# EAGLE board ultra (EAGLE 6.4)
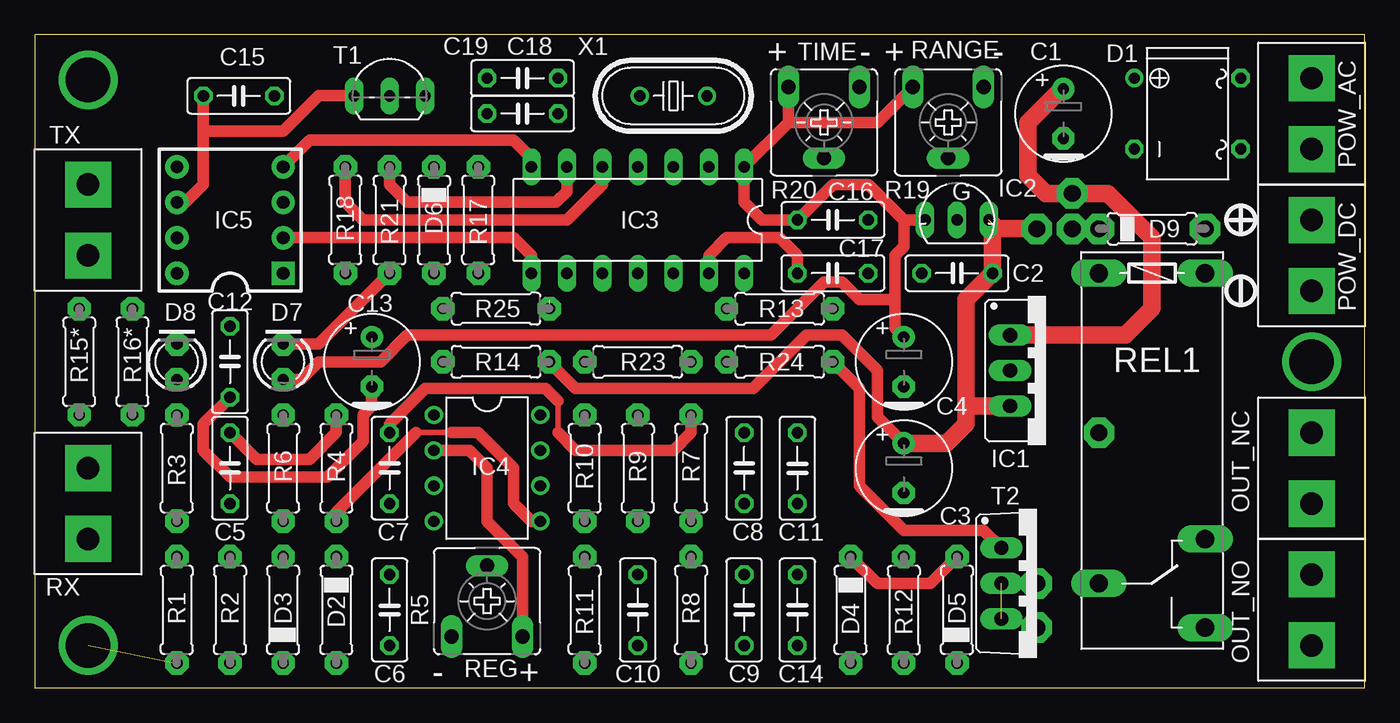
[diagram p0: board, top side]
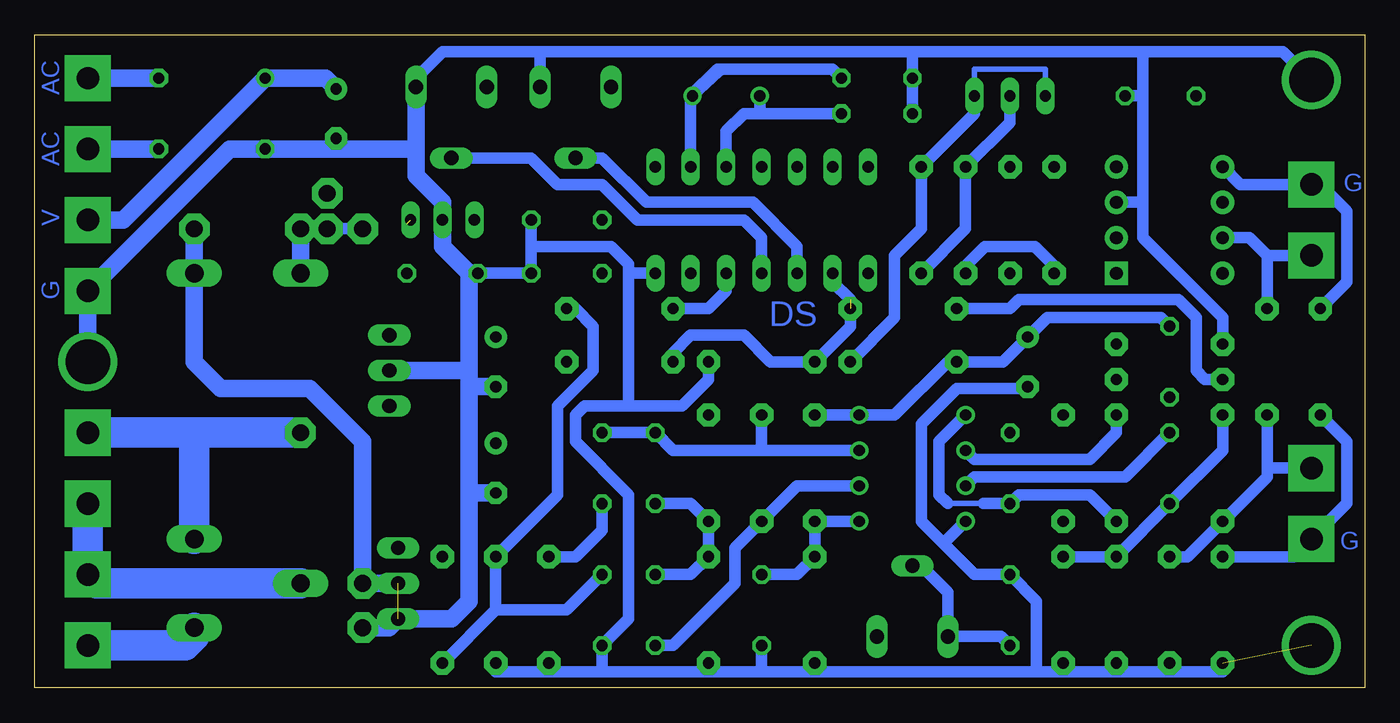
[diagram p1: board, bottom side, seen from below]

Size 95.23 x 46.79 mm. Coordinates in mm from the lower left corner, seen from the top.
Outline: 0,0 95.23,0 95.23,46.79 0,46.79 0,0
Copper layers (1*16): Top 0.035mm / dielectric 1.5mm / Bottom 0.035mm
Design rules "default": minimum track width 10mil, minimum drill 24mil, track to track 8mil, track to pad 8mil, pad to pad 8mil, via to via 8mil, smd to smd 8mil, copper to edge 40mil, drill to drill 8mil, minimum pad ring 10mil, minimum via ring 8mil, stop-mask expansion 4mil, vias tented up to drill 0mil, thermal gap 10mil

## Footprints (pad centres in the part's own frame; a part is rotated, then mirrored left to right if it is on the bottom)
E2,5-7 = drill 0.813 pad 1.6: + -1.778,0 | drill 0.813 pad 1.6 octagon: - 1.778,0
C050-025X075 = drill 0.813 octagon: 1 -2.54,0; 2 2.54,0
B-DIL = drill 0.813: + -2.54,-3.81 | drill 0.813 octagon: - 2.54,-3.81; AC1 2.54,3.81; AC2 -2.54,3.81
0207/7 = drill 0.813 pad 1.676 octagon: 1 -3.81,0; 2 3.81,0
LED3MM = drill 0.813 pad 1.676 octagon: A -1.27,0; K 1.27,0
78XXS = drill 1.016 long: GND 0,-2.54; IN -2.54,-2.54; OUT 2.54,-2.54
78LXX = drill 0.813 pad 1.27 long: GND 0,0; IN 2.286,0; OUT -2.286,0
DIL14 = drill 0.813 long: 1 -7.62,-3.81; 2 -5.08,-3.81; 3 -2.54,-3.81; 4 0,-3.81; 5 2.54,-3.81; 6 5.08,-3.81; 7 7.62,-3.81; 8 7.62,3.81; 9 5.08,3.81; 10 2.54,3.81; 11 0,3.81; 12 -2.54,3.81; 13 -5.08,3.81; 14 -7.62,3.81
DIL08 = drill 0.813 pad 1.27: 1 -3.81,-3.81; 2 -1.27,-3.81; 3 1.27,-3.81; 4 3.81,-3.81; 5 3.81,3.81; 6 1.27,3.81; 7 -1.27,3.81; 8 -3.81,3.81
MC33152 = drill 0.9 pad 1.676 square: 1 -3.81,-3.81 | drill 0.9 pad 1.676: 2 -1.27,-3.81; 3 1.27,-3.81; 4 3.81,-3.81; 5 3.81,3.81; 6 1.27,3.81; 7 -1.27,3.81; 8 -3.81,3.81
ARK2/500 = drill 1.6 pad 3.302 square: 1 -2.54,0; 2 2.54,0
CA6V = drill 1.016 long: A -2.54,-2.54; E 2.54,-2.54; S 0,2.54
G6RW = drill 1.321 long: 1 -12.7,-3.81; 2 -12.7,3.81; O 6.35,3.81; P 9.525,-3.81; S 12.7,3.81
TO92-EBC = drill 0.813 long: B 0,-1.27; C -2.54,-1.27; E 2.54,-1.27
TO220BV = drill 1.016 long: D 0,-2.54; G -2.54,-2.54; S 2.54,-2.54
HC49U70 = drill 0.813: 1 -2.413,0; 2 2.413,0

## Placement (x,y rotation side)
C1  220uF  [E2,5-7]  73.66,41.15 270 top
C2  100nF  [C050-025X075]  66.04,29.72 0 top
C3  100uF  [E2,5-7]  62.23,15.75 270 top
C4  100uF  [E2,5-7]  62.23,23.37 270 top
C5  10nF  [C050-025X075]  13.97,15.75 90 top
C6  100nF  [C050-025X075]  25.4,5.59 270 top
C7  100nF  [C050-025X075]  25.4,15.75 90 top
C8  1nF  [C050-025X075]  50.8,15.75 90 top
C9  1nF  [C050-025X075]  50.8,5.59 90 top
C10  100nF  [C050-025X075]  43.18,5.59 90 top
C11  100nF  [C050-025X075]  54.61,15.75 270 top
C12  100nF  [C050-025X075]  13.97,23.37 90 top
C13  100uF  [E2,5-7]  24.13,23.37 270 top
C14  100nF  [C050-025X075]  54.61,5.59 90 top
C15  100nF  [C050-025X075]  14.61,42.42 180 top
C16  100nF  [C050-025X075]  57.15,33.53 180 top
C17  100nF  [C050-025X075]  57.15,29.72 180 top
C18  10pF  [C050-025X075]  34.92,41.15 180 top
C19  10pF  [C050-025X075]  34.92,43.69 180 top
D1  [B-DIL]  82.55,41.15 270 top
D2  BAT43  [0207/7]  21.59,5.59 90 top
D3  BAT43  [0207/7]  17.78,5.59 90 top
D4  BAT43  [0207/7]  58.42,5.59 90 top
D5  BAT43  [0207/7]  66.04,5.59 90 top
D6  DZ9V1  [0207/7]  28.57,33.53 270 top
D7  [LED3MM]  17.78,23.37 90 top
D8  [LED3MM]  10.16,23.37 90 top
D9  BAT43  [0207/7]  80.01,32.89 180 top
IC1  LM2940-12  [78XXS]  72.39,22.73 270 top
IC2  78L05  [78LXX]  66.04,33.53 0 top
IC3  ATTINY24  [DIL14]  43.18,33.53 180 top
IC4  TL072  [DIL08]  32.38,15.75 270 top
IC5  MC33152  [MC33152]  13.97,33.53 90 top
OUT_NC  ARK2ARK2/500  [ARK2/500]  91.44,15.75 90 top
OUT_NO  ARK2ARK2/500  [ARK2/500]  91.44,5.59 90 top
POW_AC  [ARK2/500]  91.44,41.15 270 top
POW_DC  ARK2ARK2/500  [ARK2/500]  91.44,30.99 270 top
R1  100R  [0207/7]  10.16,5.59 90 top
R2  1M  [0207/7]  13.97,5.59 90 top
R3  2k  [0207/7]  10.16,15.75 270 top
R4  1M  [0207/7]  21.59,15.75 270 top
R5  100k  [CA6V]  32.38,6.22 0 top
R6  1M  [0207/7]  17.78,15.75 270 top
R7  510R  [0207/7]  46.99,15.75 270 top
R8  510R  [0207/7]  46.99,5.59 90 top
R9  68k  [0207/7]  43.18,15.75 90 top
R10  2k  [0207/7]  39.37,15.75 90 top
R11  2k  [0207/7]  39.37,5.59 90 top
R12  2k  [0207/7]  62.23,5.59 90 top
R13  10k  [0207/7]  53.34,27.18 0 top
R14  100R  [0207/7]  33.02,23.37 180 top
R15*  0R  [0207/7]  3.18,23.37 90 top
R16*  0R  [0207/7]  6.99,23.37 90 top
R17  10k  [0207/7]  31.75,33.53 270 top
R18  2k  [0207/7]  22.23,33.53 90 top
R19  100k  [CA6V]  65.41,40.51 180 top
R20  100k  [CA6V]  56.51,40.51 180 top
R21  2k  [0207/7]  25.4,33.53 90 top
R23  10k  [0207/7]  43.18,23.37 0 top
R24  100R  [0207/7]  53.34,23.37 0 top
R25  2k  [0207/7]  33.02,27.18 0 top
REL1  JQX68-12V  [G6RW]  80.01,17.02 270 top
RX  RX  [ARK2/500]  3.81,13.21 270 top
T1  BC557  [TO92-EBC]  25.4,43.69 0 top
T2  IRL540  [TO220BV]  71.76,7.49 270 top
TX  TX  [ARK2/500]  3.81,33.53 90 top
X1  16MHz  [HC49U70]  45.72,42.42 180 top

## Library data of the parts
C1-C19 D2-D6 D9 R1-R4 R6-R14 R15* R16* R17 R18 R21 R23-R25 = rcl
D1 = rectifier
D7 D8 = led
IC1 IC2 = v-reg
IC3 = avr-7
IC4 = linear
IC5 = MC33152
OUT_NC OUT_NO POW_AC POW_DC RX TX = dimmer
R5 R19 R20 = pot
REL1 = relay; OC_FARNELL: unknown; OC_NEWARK: unknown
T1 = transistor-pnp
T2 = transistor-power
X1 = crystal; OC_FARNELL: unknown; OC_NEWARK: unknown

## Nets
!PULSE: IC3.7 IC5.4
AOUT: IC3.12 R13.1
DEN: IC3.5 R18.2
GND: C1.- C2.1 C3.- C4.- C6.1 C10.1 C12.1 C13.- C14.1 C15.1 C16.1 C17.1 C18.2 C19.2 D1.- D2.1 D3.1 D4.1 D8.K IC1.GND IC2.GND IC3.14 IC4.4 IC5.3 POW_DC.2 R1.1 R2.1 R8.1 R11.1 R12.1 R19.A R20.A R23.2 T2.S
N$1: R2.2 R3.2 R16*.1 RX.1
N$2: R1.2 R15*.1 RX.2
N$3: C5.1 D2.2 D3.2 R3.1
N$4: C6.2 R5.A R5.S
N$5: C5.2 IC4.3 R4.1
N$6: IC4.2 R5.E R6.1
N$7: C7.1 IC4.1 R6.2
N$8: C7.2 R7.1
N$9: C8.1 C9.2 R7.2 R8.2
N$10: C9.1 IC4.6 R9.1
N$11: C8.2 C11.1 IC4.7 R9.2
N$12: C11.2 D4.2 D5.2
N$13: C14.2 D5.1 R12.2 R13.2
N$14: C12.2 C13.+ IC4.8 R10.2 R14.2
N$15: D6.1 R17.2 T1.B
N$16: IC5.5 R15*.2 TX.2
N$17: IC5.7 R16*.2 TX.1
N$18: C17.2 IC3.13
N$19: D6.2 R18.1
N$20: C15.2 IC5.6 T1.C
N$21: C19.1 IC3.2 X1.1
N$22: C18.1 IC3.3 X1.2
N$24: IC3.6 R21.2
N$25: D7.K R21.1
N$27: R24.2 T2.G
N$28: OUT_NC.2 REL1.O
N$29: D8.A R25.1
N$31: D1.AC2 POW_AC.1
N$32: D1.AC1 POW_AC.2
N$33: OUT_NC.1 OUT_NO.2 REL1.P
N$34: OUT_NO.1 REL1.S
N$37: C1.+ D1.+ IC1.IN POW_DC.1
N$38: D9.1 REL1.2 T2.D
OUT: IC3.9 R23.1 R24.1 R25.2
PULSE: IC3.8 IC5.2
RANGE: IC3.11 R19.S
TIME: IC3.10 R20.S
VA2: C10.2 IC4.5 R4.2 R10.1 R11.2
VCC: C2.2 C3.+ D9.2 IC1.OUT IC2.IN R14.1 R17.1 REL1.1 T1.E
VDD: C4.+ C16.2 D7.A IC2.OUT IC3.1 R19.E R20.E

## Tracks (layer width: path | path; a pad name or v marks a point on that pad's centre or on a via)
!PULSE
  Top 0.813: IC5.4 19.68,39.24 34.29,39.24 35.56,37.97 IC3.7
AOUT
  Bottom 0.813: IC3.12 45.72,28.45 46.99,27.18 R13.1
DEN
  Top 0.813: IC3.5 40.64,36.07 38.1,33.53 23.5,33.53 22.23,34.8 R18.2
GND  (via drill 3.2)  (1 unrouted)
  Top 0.813: C12.1 12.07,18.92 12.07,17.02 13.97,15.11 20.96,15.11 23.5,17.65 23.5,19.56 24.13,20.19 C13.-
  Bottom 0.813: 15.88,34.8 15.88,32.26 10.16,26.54 D8.K | 15.88,34.8 15.88,42.42 | 15.88,42.42 15.88,45.59 | 15.88,45.59 32.38,45.59 | 32.38,45.59 59.05,45.59 | 59.05,45.59 66.04,45.59 67.95,43.69 R19.A | C15.1 15.88,42.42 | IC5.3 15.88,34.8 | 32.38,45.59 C19.2 C18.2 | v3.81,43.56 5.84,45.59 15.88,45.59 | 21.59,1.14 17.78,1.14 | 17.78,1.14 13.97,1.14 | 13.97,1.14 10.16,1.14 R1.1 | 58.42,1.14 62.23,1.14 R12.1 | 58.42,1.14 54.61,1.14 | 54.61,1.14 46.99,1.14 | 46.99,1.14 43.18,1.14 | 43.18,1.14 39.37,1.14 | 39.37,1.14 23.5,1.14 | 23.5,1.14 21.59,1.14 | R11.1 39.37,1.14 | C10.1 43.18,1.14 | R2.1 13.97,1.14 | D3.1 17.78,1.14 | D2.1 21.59,1.14 | 23.5,1.14 23.5,6.22 C6.1 27.94,8.13 30.16,10.35 | R8.1 46.99,1.14 | 54.61,1.14 C14.1 52.7,4.95 52.7,13.84 56.51,17.65 56.51,19.56 55.88,20.19 52.7,20.19 | D4.1 58.42,1.14 | R23.2 46.99,22.1 48.89,20.19 52.7,20.19 | IC3.14 52.7,29.72 | 52.7,29.72 52.7,20.19 | 52.7,29.72 52.7,30.35 53.97,31.62 59.56,31.62 59.69,31.5 | R20.A 59.05,45.59 | C13.- 24.13,21.46 29.21,21.46 31.75,18.92 31.75,11.94 30.16,10.35 | IC4.4 30.16,10.35 | C2.1 C17.1 59.69,31.5 | C16.1 59.69,31.5
  Bottom 1.27: 67.95,38.61 67.95,36.7 66.04,34.8 IC2.GND 66.04,31.62 64.14,29.72 | 67.95,38.61 R19.A | T2.S 65.41,4.95 64.14,6.22 64.14,13.84 | 73.66,38.61 D1.- 81.28,38.61 POW_DC.2 v91.44,23.37 | 73.66,38.61 67.95,38.61 | C1.- 73.66,38.61 | 64.14,13.84 64.14,21.46 | 64.14,21.46 64.14,22.73 | 64.14,22.73 64.14,29.72 | C2.1 64.14,29.72 | C4.- 64.01,21.59 64.14,21.46 | IC1.GND 64.14,22.73 | C3.- 64.01,13.97 64.14,13.84
  other vias: 3.81,3.05
N$1
  Bottom 0.813: R2.2 12.7,9.4 R3.2 6.99,15.11 6.99,15.75 | R16*.1 6.99,15.75 | RX.1 6.99,15.75
N$2
  Bottom 0.813: R15*.1 1.27,17.65 1.27,13.21 RX.2 5.08,9.4 R1.2
N$3
  Bottom 0.813: D2.2 D3.2 C5.1 10.16,17.02 R3.1
N$4
  Bottom 0.813: C6.2 26.04,3.68 R5.A 29.84,6.86 31.75,8.76 R5.S
N$5
  Top 0.813: R4.1 21.59,18.29 19.68,16.38 15.88,16.38 C5.2
  Bottom 0.813: IC4.3 27.94,15.11 17.14,15.11 C5.2
N$6
  Top 0.813: IC4.2 31.11,17.02 32.38,15.75 32.38,11.94 34.92,9.4 R5.E
  Bottom 0.813: R6.1 17.78,18.29 19.68,16.38 27.94,16.38 IC4.2
N$7
  Bottom 0.406: 29.84,13.21 27.3,13.21
  Bottom 0.813: R6.2 19.68,13.84 24.77,13.84 C7.1 27.3,13.21 | IC4.1 30.48,17.65 30.48,13.84 29.84,13.21
N$8
  Top 0.406: 37.46,20.57 37.46,18.29
  Top 0.813: C7.2 25.4,18.92 27.94,21.46 36.58,21.46 37.46,20.57 | 37.46,18.29 38.73,17.02 45.72,17.02 46.99,18.29 R7.1
N$9
  Bottom 0.813: C8.1 48.26,13.21 R7.2 R8.2 48.26,8.13 C9.2
N$10
  Bottom 0.813: IC4.6 40.64,14.48 R9.1 45.08,10.03 45.08,7.49 49.53,3.05 C9.1
N$11
  Bottom 0.813: IC4.7 43.18,17.02 | 43.18,17.02 49.53,17.02 C8.2 C11.1 | R9.2 43.18,17.02
N$12
  Top 0.813: D4.2 60.32,7.49 64.14,7.49 D5.2
  Bottom 0.813: C11.2 54.61,11.3 56.51,9.4 D4.2
N$13
  Bottom 0.813: C14.2 57.15,5.59 62.23,5.59 | 62.23,5.59 D5.1 | 62.23,5.59 R12.2 57.78,13.84 57.78,20.19 55.24,22.73 55.24,25.91 56.51,27.18 R13.2
N$14
  Bottom 0.813: R10.2 IC4.8 33.65,19.56 29.84,23.37 R14.2 25.91,23.37 C13.+ 22.73,26.54 14.61,26.54 C12.2
N$15
  Bottom 0.813: T1.B 25.4,40.51 D6.1 28.57,32.89 R17.2
N$16
  Bottom 0.813: R15*.2 1.27,29.08 1.27,34.16 3.18,36.07 TX.2 8.89,36.07 IC5.5
N$17
  Bottom 0.813: R16*.2 6.99,30.99 | IC5.7 8.26,32.26 6.99,30.99 | TX.1 6.99,30.99
N$18
  Top 0.813: C17.2 54.61,30.99 53.34,32.26 49.53,32.26 48.26,30.99 IC3.13
N$19
  Bottom 0.813: R18.1 22.23,30.23 23.62,31.62 27.18,31.62 28.57,30.23 D6.2
N$20
  Top 0.813: IC5.6 10.79,34.8 12.07,36.07 12.07,39.88 | 12.07,39.88 C15.2 | T1.C 20.32,42.42 17.78,39.88 12.07,39.88
  Bottom 0.406: T1.C 22.86,44.32 27.94,44.32 27.94,42.54
N$21
  Bottom 0.813: C19.1 38.1,44.32 46.35,44.32 | 46.35,44.32 48.26,42.42 IC3.2 | X1.1 46.23,44.2 46.35,44.32
N$22
  Bottom 0.813: IC3.3 45.72,39.88 44.45,41.15 43.18,41.15 | 43.18,41.15 C18.1 | X1.2 43.31,41.27 43.18,41.15
N$23  (via drill 1.2 pad 2.18)
  other vias: 83.82,32.89
N$24
  Top 0.813: IC3.6 38.1,35.56 37.34,34.8 26.67,34.8 25.4,36.07 R21.2
N$25
  Top 0.813: R21.1 20.32,24.64 D7.K
N$27
  Top 0.813: R24.2 59.05,21.46 59.05,14.48 62.23,11.3 67.95,11.3 T2.G
N$28  (via drill 1.2 pad 2.18)
  Bottom 2.184: v76.2,18.29 83.82,18.29 | 83.82,18.29 OUT_NC.2 | REL1.O 83.82,18.29
N$29
  Bottom 0.813: D8.A 11.43,22.1 12.07,22.73 12.07,26.54 13.34,27.81 24.77,27.81 25.4,27.18 R25.1
N$31
  Bottom 1.27: POW_AC.1 D1.AC2
N$32
  Bottom 1.27: POW_AC.2 D1.AC1
N$33
  Bottom 2.184: OUT_NC.1 OUT_NO.2 90.81,7.49 REL1.P
N$34
  Bottom 2.184: REL1.S 83.82,3.68 84.45,3.05 OUT_NO.1
N$37  (via drill 1.2 pad 2.18)
  Top 1.27: IC1.IN 78.11,25.27 80.01,27.18 80.01,32.26 76.84,35.43 v74.3,35.43 72.39,35.43 71.12,36.7 71.12,40.51 73.53,42.93 C1.+
  Bottom 1.27: C1.+ 74.42,43.69 D1.+ 88.9,33.53 POW_DC.1
N$38  (via drill 1.2 pad 2.18)  (1 unrouted)
  Bottom 1.27: v71.76,4.32 69.85,4.32 69.22,4.95 | T2.D v71.76,7.49 71.76,17.65 75.56,21.46 81.92,21.46 83.82,23.37 REL1.2 D9.1
OUT  (1 unrouted)
  Bottom 0.813: IC3.9 38.1,29.08 36.83,27.81 36.83,25.91 R23.1 42.54,23.37 44.45,25.27 48.26,25.27 49.53,24 R24.1
PULSE
  Top 0.813: IC5.2 34.29,32.26 35.56,30.99 IC3.8
RANGE
  Bottom 0.813: R19.S 59.69,37.97 57.78,36.07 54.61,36.07 52.07,33.53 44.45,33.53 43.18,32.26 IC3.11
TIME
  Bottom 0.813: IC3.10 40.64,31.62 43.81,34.8 51.43,34.8 54.61,37.97 R20.S
VA2
  Top 0.406: 29.84,18.29 27.3,18.29
  Top 0.813: IC4.5 35.56,11.94 34.29,13.21 34.29,15.75 31.75,18.29 29.84,18.29 | 27.3,18.29 21.59,12.57 R4.2
  Bottom 0.813: C10.2 40.64,8.13 R11.2 R10.1 IC4.5
VCC  (via drill 1.2 pad 2.18)  (1 unrouted)
  Top 0.813: R14.1 38.73,21.46 51.43,21.46 55.24,25.27 57.78,25.27 60.32,22.73 60.32,19.43 C3.+
  Top 1.27: IC1.OUT 66.67,20.19 | 66.67,20.19 66.67,27.81 C2.2 68.58,32.89 | C3.+ 65.28,17.53 66.67,18.92 66.67,20.19 | 68.58,32.89 68.58,33.27 | v71.76,32.89 68.58,32.89
  Bottom 0.813: v74.3,32.89 v71.76,32.89 | T1.E 27.94,41.15 R17.1 31.75,32.89 33.65,30.99 33.65,26.54 R14.1
  Bottom 1.27: v74.3,32.89 D9.2 REL1.1
  other vias: 76.2,32.89
VDD
  Top 0.813: 53.97,40.51 IC3.1 50.8,34.8 52.07,33.53 C16.2 57.15,36.07 59.69,36.07 62.23,33.53 | 53.97,40.51 60.32,40.51 R19.E | R20.E 53.97,40.51 | IC2.OUT 62.23,33.53 | 62.23,33.53 62.23,31.62 61.59,30.99 61.59,27.69 | 61.59,27.69 61.59,25.78 C4.+ | D7.A 19.05,22.1 20.32,23.37 24.77,23.37 26.67,25.27 52.7,25.27 56.51,29.08 57.78,29.08 59.05,27.81 61.47,27.81 61.59,27.69

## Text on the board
Bottom: AC | AC | G | V | G | DS | G
tPlace: TIME | RANGE | + | - | + | - | - | REG | +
